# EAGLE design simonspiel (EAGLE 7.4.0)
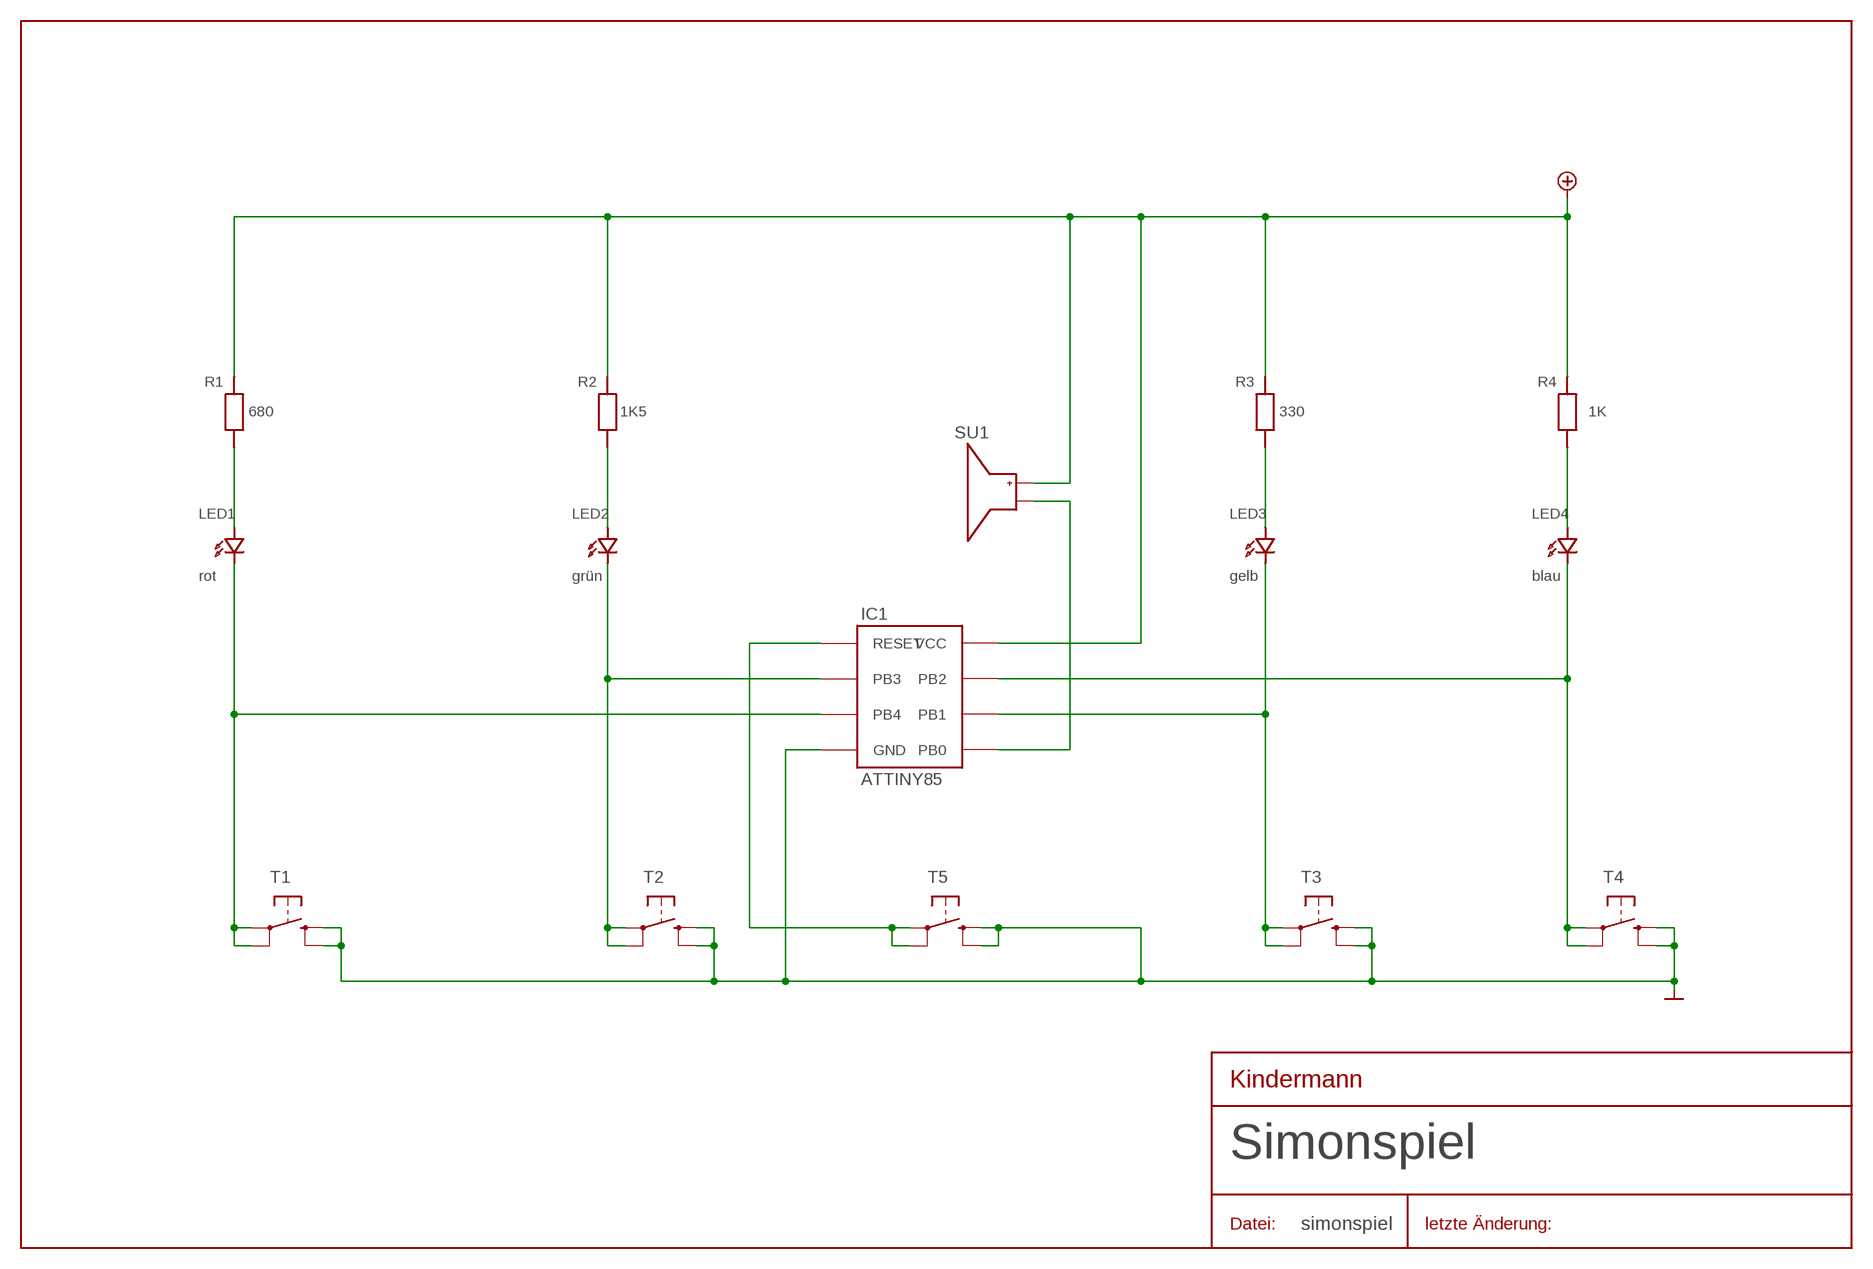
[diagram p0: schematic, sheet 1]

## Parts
GND  GND  [GND]
IC1  ATTINY85  [ATTINY85]
LED1  LED_3MM_ROT  [LED_ROT_LANG_3MM]
LED2  LED_3MM_GRUEN  [LED_GRUEN_LANG_3MM]
LED3  LED_3MM_GELB  [LED_GELB_LANG_3MM]
LED4  LED_3MM_BLAU  [LED_BLAU_LANG_3MM]
R1  WID_680  [WIDERSTAND_680]
R2  WID_1K5  [WIDERSTAND_1K5]
R3  WID_330  [WIDERSTAND_330]
R4  WID_1K  [WIDERSTAND_1K]
SU1  SUMMER  [SUMMER]
T1  OMRON_TASTER  [OMRON_TASTER_2]
T2  OMRON_TASTER  [OMRON_TASTER_2]
T3  OMRON_TASTER  [OMRON_TASTER_2]
T4  OMRON_TASTER  [OMRON_TASTER_2]
T5  MICROTASTER  [MICROTASTER]
VCC  VCC  [VCC]

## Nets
GND: GND.GND IC1.4(GND) T1.1(S1) T1.2(S) T2.1(S1) T2.2(S) T3.1(S1) T3.2(S) T4.1(S1) T4.2(S) T5.1(S1) T5.2(S)
N$1: LED1.1(A) R1.1
N$2: LED2.1(A) R2.1
N$3: IC1.3(PB4) LED1.2(K) T1.3(P1) T1.4(P)
N$4: LED3.1(A) R3.1
N$6: IC1.7(PB2) LED4.2(K) T4.3(P1) T4.4(P)
N$8: IC1.5(PB0) SU1.2
N$9: LED4.1(A) R4.1
N$11: IC1.1(RESET) T5.3(P1) T5.4(P)
N$12: IC1.6(PB1) LED3.2(K) T3.3(P1) T3.4(P)
N$15: IC1.2(PB3) LED2.2(K) T2.3(P1) T2.4(P)
VCC: IC1.8(VCC) R1.2 R2.2 R3.2 R4.2 SU1.1 VCC.VCC

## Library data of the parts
GND = simon-profil-9:GND
IC1 = simon-profil-9:ATTINY85
LED1 = simon-profil-9:LED_3MM_ROT
LED2 = simon-profil-9:LED_3MM_GRUEN
LED3 = simon-profil-9:LED_3MM_GELB
LED4 = simon-profil-9:LED_3MM_BLAU
R1 = simon-profil-9:WID_680
R2 = simon-profil-9:WID_1K5
R3 = simon-profil-9:WID_330
R4 = simon-profil-9:WID_1K
SU1 = simon-profil-9:SUMMER
T1-T4 = simon-profil-9:OMRON_TASTER
T5 = simon-profil-9:MICROTASTER
VCC = simon-profil-9:VCC

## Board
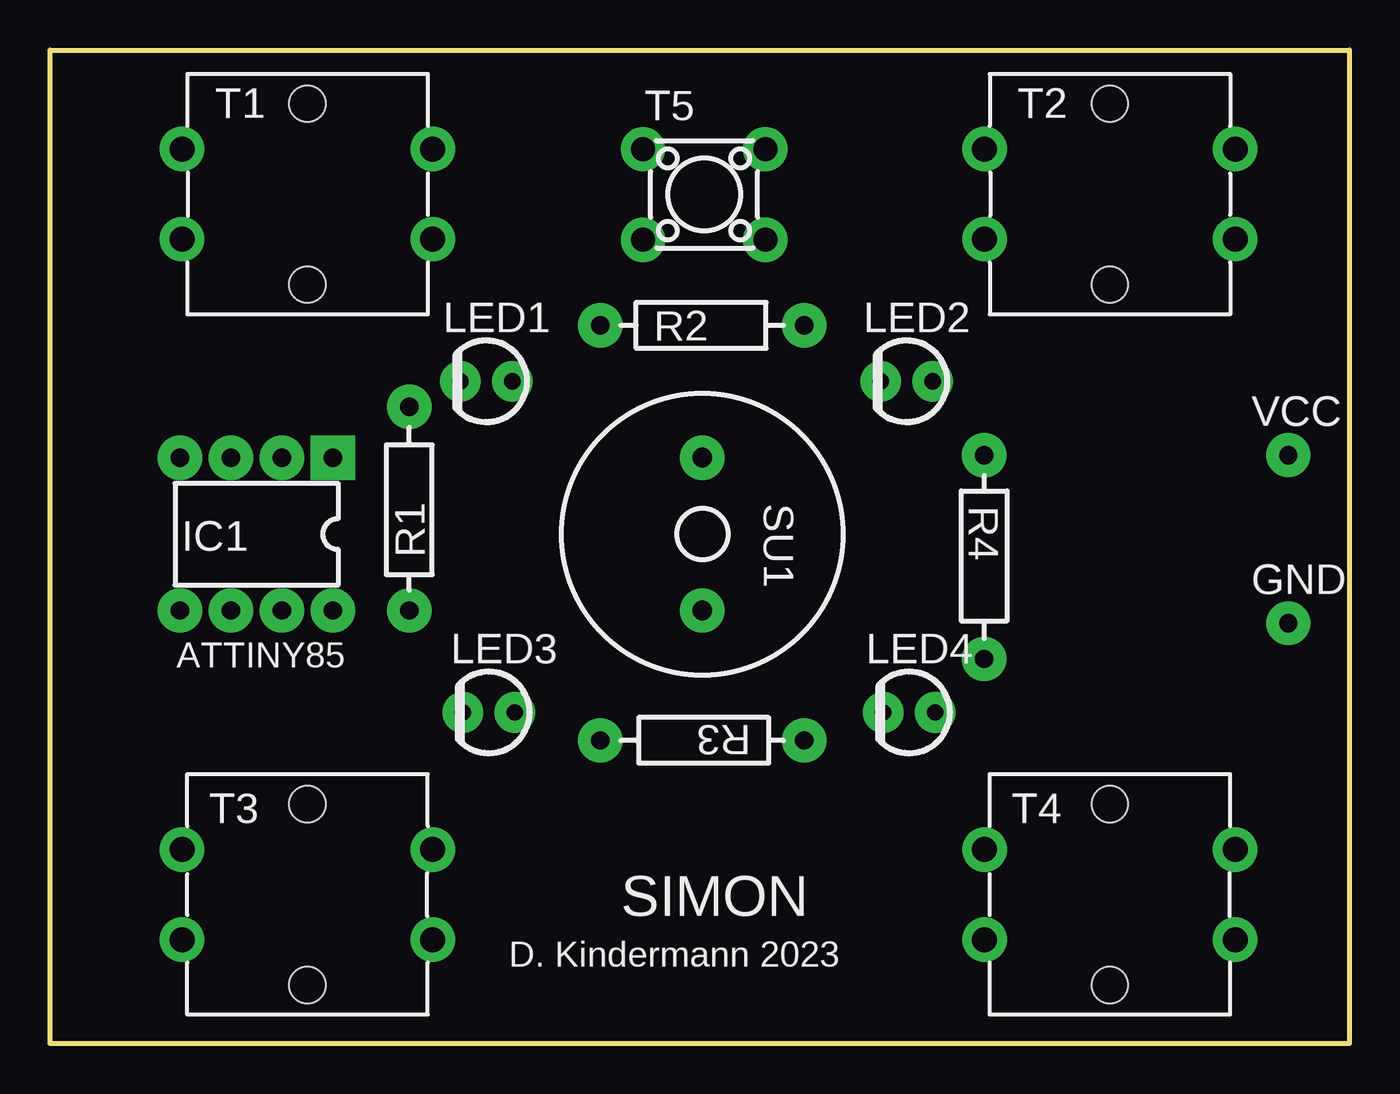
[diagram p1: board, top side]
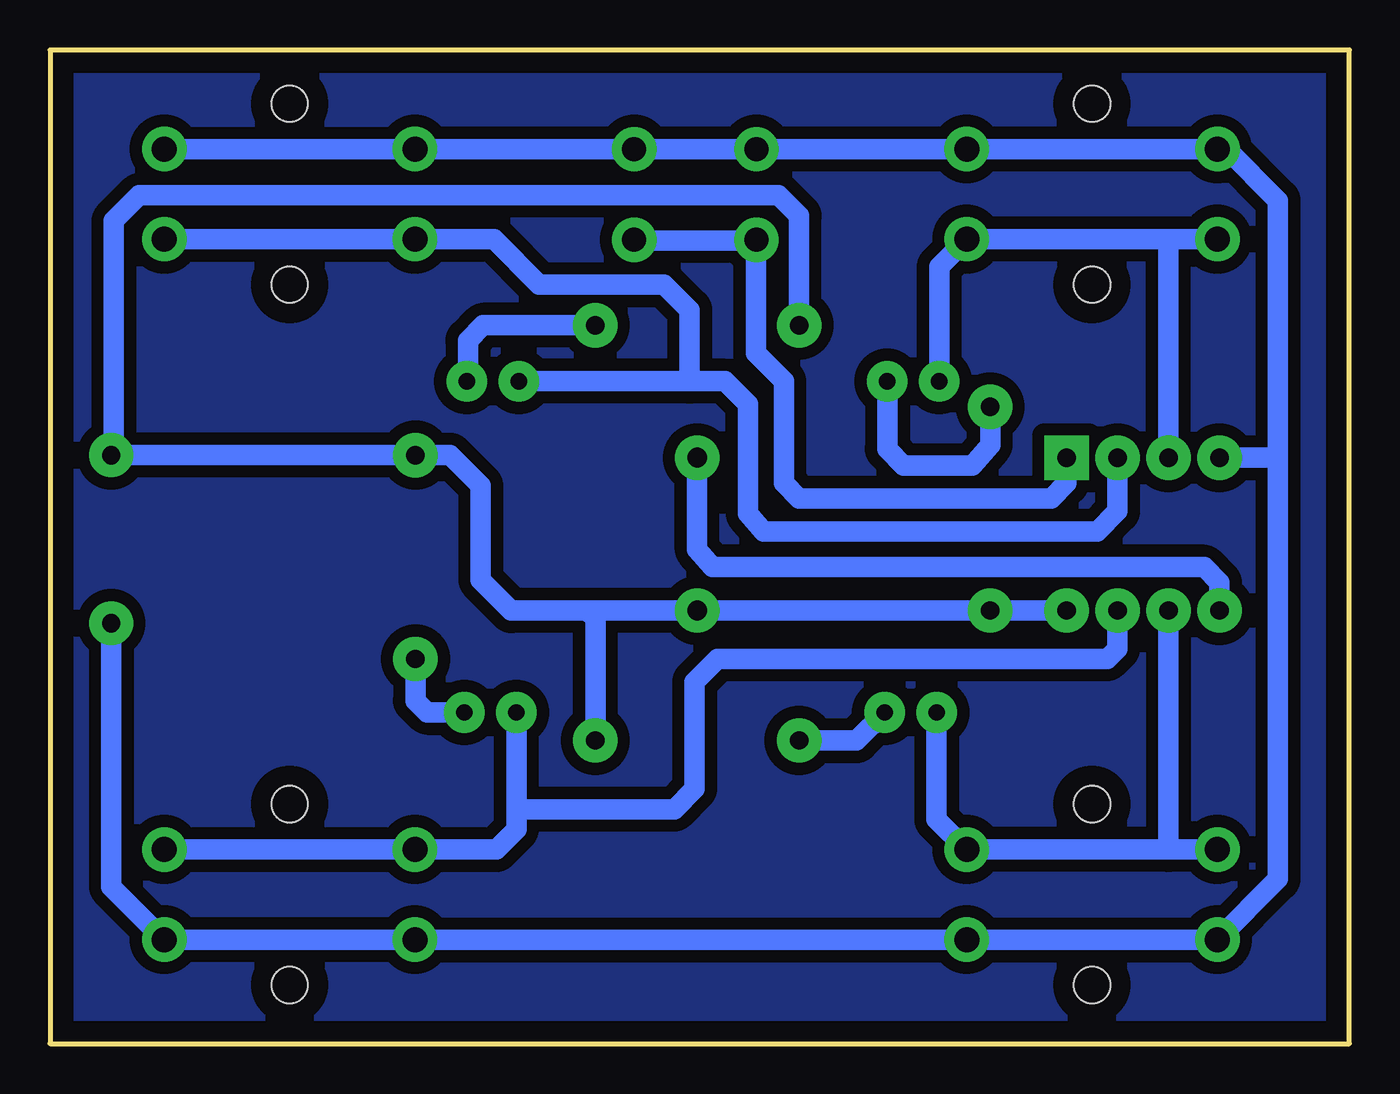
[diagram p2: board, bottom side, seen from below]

Size 64.77 x 49.53 mm. Coordinates in mm from the lower left corner, seen from the top.
Outline: 0,49.53 64.77,49.53 64.77,0 0,0 0,49.53
Copper layers (1*16): Top 0.035mm / dielectric 1.5mm / Bottom 0.035mm
Design rules "default": minimum track width 10mil, minimum drill 0.6mm, track to track 8mil, track to pad 8mil, pad to pad 8mil, via to via 8mil, smd to smd 8mil, copper to edge 40mil, drill to drill 8mil, minimum pad ring 10mil, minimum via ring 8mil, stop-mask expansion 4mil, vias tented up to drill 0mil, thermal gap 10mil

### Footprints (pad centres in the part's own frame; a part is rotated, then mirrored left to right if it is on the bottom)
GND = drill 0.914 pad 2.184: GND 0,0
ATTINY85 = drill 0.914 pad 2.21 square: 1 -3.81,3.81 | drill 0.914 pad 2.21: 2 -3.81,1.27; 3 -3.81,-1.27; 4 -3.81,-3.81; 5 3.81,-3.81; 6 3.81,-1.27; 7 3.81,1.27; 8 3.81,3.81
LED_ROT_LANG_3MM = drill 0.813 pad 2.032: 1 2.591,0; 2 0,0
LED_GRUEN_LANG_3MM = drill 0.813 pad 2.032: 1 2.591,0; 2 0,0
LED_GELB_LANG_3MM = drill 0.813 pad 2.032: 1 2.591,0; 2 0,0
LED_BLAU_LANG_3MM = drill 0.813 pad 2.032: 1 2.591,0; 2 0,0
WIDERSTAND_680 = drill 0.914 pad 2.21: 1 5.08,0; 2 -5.08,0
WIDERSTAND_1K5 = drill 0.914 pad 2.21: 1 5.08,0; 2 -5.08,0
WIDERSTAND_330 = drill 0.914 pad 2.21: 1 5.08,0; 2 -5.08,0
WIDERSTAND_1K = drill 0.914 pad 2.21: 1 5.08,0; 2 -5.08,0
SUMMER = drill 0.991 pad 2.21: 1 3.81,0; 2 -3.81,0
OMRON_TASTER_2 = drill 1.245 pad 2.21: 1 6.248,-2.438; 2 -6.248,-2.438; 3 6.248,2.057; 4 -6.248,2.057 | hole 1.803: 0,-4.699; 0,4.318
MICROTASTER = drill 1.194 pad 2.21: 1 -3.048,2.261; 2 3.048,2.261; 3 -3.048,-2.261; 4 3.048,-2.261
VCC = drill 0.914 pad 2.184: VCC 0,0

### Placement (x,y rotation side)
GND  61.72,20.95 0 top
IC1  10.29,25.4 270 top
LED1  20.45,33.02 0 top
LED2  41.4,33.02 0 top
LED3  20.57,16.51 0 top
LED4  41.53,16.51 0 top
R1  17.91,26.67 90 top
R2  32.51,35.81 0 top
R3  32.51,15.11 180 top
R4  46.56,24.26 270 top
SU1  32.51,25.4 270 top
T1  12.83,42.16 180 top
T2  52.83,42.16 180 top
T3  12.83,7.62 0 top
T4  52.83,7.62 0 top
T5  32.6,42.33 0 top
VCC  61.72,29.34 0 top

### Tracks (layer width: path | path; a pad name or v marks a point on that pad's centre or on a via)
GND
  Bottom 1.016: T2.2 T2.1 T5.2 T5.1 T1.2 T1.1 6.12,44.6 3.56,42.04 3.56,29.34 | 3.56,29.34 3.56,8.2 T3.2 T3.1 T4.2 T4.1 61.72,7.82 GND.GND | IC1.4 3.68,29.21 3.56,29.34
N$1
  Bottom 1.016: LED1.1 23.04,29.64 22.23,28.83 18.8,28.83 17.91,29.84 R1.1
N$2
  Bottom 1.016: R2.1 43.18,35.81 43.94,35.05 43.94,33.07 LED2.1
N$3
  Bottom 1.016: T1.3 9.14,40.11 | 9.14,40.11 T1.4 20.45,38.73 LED1.2 | IC1.3 9.02,39.98 9.14,40.11
N$4
  Bottom 1.016: R3.1 24.56,15.11 LED3.1
N$5
  pour Bottom (isolate 0.61): 0,0 64.77,0 64.77,49.53 0,49.53
N$6
  Bottom 1.016: 41.53,11.81 41.53,10.67 42.52,9.68 T4.4 T4.3 | 41.53,11.81 LED4.2 | IC1.7 11.56,19.68 12.06,19.18 31.5,19.18 32.64,18.03 32.64,12.7 33.66,11.68 41.4,11.68 41.53,11.81
N$8
  Bottom 1.016: IC1.5 6.48,22.99 7.24,23.75 31.75,23.75 32.51,24.64 SU1.2
N$9
  Bottom 1.016: R4.1 46.56,17.09 45.97,16.51 LED4.1
N$11
  Bottom 1.016: IC1.1 14.1,27.94 14.86,27.18 27.43,27.18 28.19,27.94 28.19,33.02 29.59,34.42 29.59,40.04 | 29.59,40.04 T5.3 | 29.59,40.04 35.62,40.04 T5.4
N$12
  Bottom 1.016: LED3.2 20.57,11.18 T3.3 9.02,9.68 | T3.4 9.02,9.68 | IC1.6 9.02,9.68
N$15
  Bottom 1.016: T2.4 T2.3 42.65,40.11 40.39,37.85 34.16,37.85 32.89,36.58 32.89,33.02 | IC1.2 11.56,26.54 12.57,25.53 29.21,25.53 29.97,26.42 29.97,31.88 31.11,33.02 32.89,33.02 | 32.89,33.02 LED2.2
VCC
  Bottom 1.016: IC1.8 R1.2 SU1.1 37.97,21.59 | 37.97,21.59 41.78,21.59 43.31,23.11 43.31,27.81 44.83,29.34 R4.2 VCC.VCC 61.59,29.46 61.59,41.02 60.33,42.29 28.45,42.29 27.43,41.27 R2.2 | R3.2 37.59,21.21 37.97,21.59

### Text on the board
tPlace: SIMON | D. Kindermann 2023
